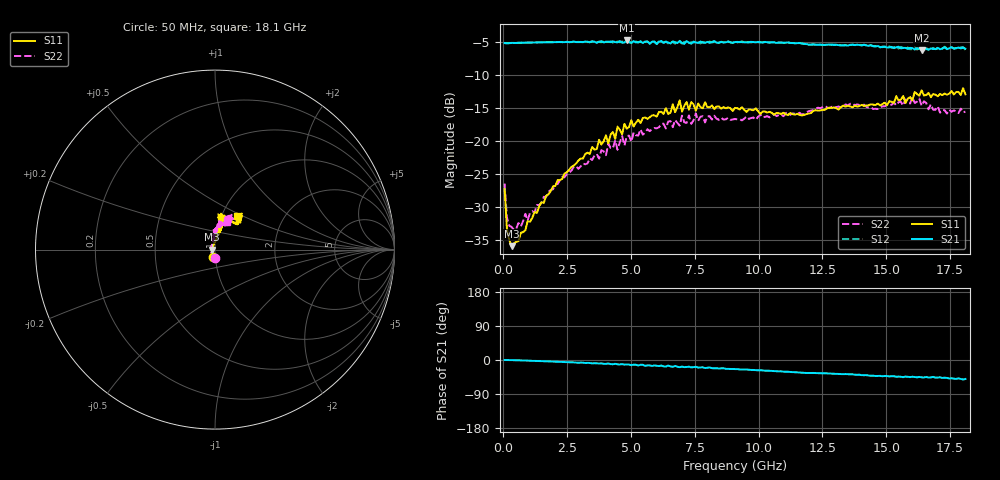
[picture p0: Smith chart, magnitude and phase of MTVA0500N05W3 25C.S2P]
! Network Analyzer HP8720D.06.14 Serial No. US36140669
!  8 Jul 2005  08:56:46
! Frequency  S11  S21  S12  S22
# HZ  S  DB R 50
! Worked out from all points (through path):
!   201 points, 50 MHz to 18.1 GHz, reference 50 ohm
!   highest |S21| = -4.81 dB at 4.833 GHz (marker M1); lowest = -6.3 dB at 16.39 GHz (marker M2)
!   group delay of S21, straight-line fit = 8.03 ps
!   lowest |S11| = -35.9 dB at 320.8 MHz (marker M3), VSWR 1.03, Z = 48.4 - j0.0679 ohm
!   |S11| at or under -10 dB: start of sweep to end of sweep
!   |S22| runs from -33.4 to -13.4 dB; largest |S21 - S12| = 0.026
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5e7  -27.26 -107.2  -5.19 0.0  -5.22 0.1  -26.43 -93.3
1.4025e8  -33.20 -135.2  -5.24 -0.1  -5.22 -0.1  -31.55 -140.8
3.2075e8  -35.87 -177.5  -5.18 -0.3  -5.20 -0.3  -32.96 -176.6
9.525e8  -32.10 118.1  -5.12 -1.6  -5.13 -1.6  -31.99 134.8
2.12575e9  -25.92 86.1  -5.05 -4.9  -5.06 -4.7  -26.49 101.6
3.1185e9  -22.63 82.1  -5.06 -7.0  -5.07 -7.4  -23.39 99.3
4.021e9  -19.12 79.5  -4.99 -10.3  -5.06 -9.4  -22.13 92.0
4.382e9  -19.65 77.5  -5.06 -9.9  -5.03 -11.3  -19.90 92.4
4.47225e9  -17.82 73.5  -5.09 -11.4  -4.97 -10.4  -21.31 95.3
4.83325e9  -18.14 82.3  -4.81 -11.8  -5.00 -12.8  -19.26 83.6
6.09675e9  -15.62 76.5  -4.99 -16.0  -4.92 -15.7  -17.92 83.3
6.7285e9  -15.63 82.9  -5.07 -15.6  -5.29 -16.7  -16.81 77.9
6.909e9  -13.86 80.5  -4.87 -19.1  -5.03 -17.5  -17.66 76.8
6.99925e9  -15.54 80.2  -5.19 -17.3  -5.28 -19.3  -16.16 78.1
7.17975e9  -14.11 84.8  -4.90 -18.5  -5.18 -17.7  -17.25 73.3
7.54075e9  -15.41 76.7  -5.11 -17.9  -4.95 -20.4  -15.84 81.6
9.075e9  -14.99 81.0  -5.04 -23.9  -5.02 -23.9  -16.67 72.3
1.21435e10  -15.46 68.6  -5.42 -34.1  -5.38 -34.3  -15.33 69.9
1.512175e10  -13.96 49.1  -5.86 -43.4  -5.69 -42.8  -14.58 71.0
1.602425e10  -13.86 53.4  -5.96 -44.0  -6.12 -46.4  -13.36 64.6
1.638525e10  -12.33 51.3  -6.26 -45.8  -6.06 -44.7  -14.69 63.0
1.81e10  -12.94 56.9  -6.04 -50.0  -6.23 -51.0  -15.55 65.4
